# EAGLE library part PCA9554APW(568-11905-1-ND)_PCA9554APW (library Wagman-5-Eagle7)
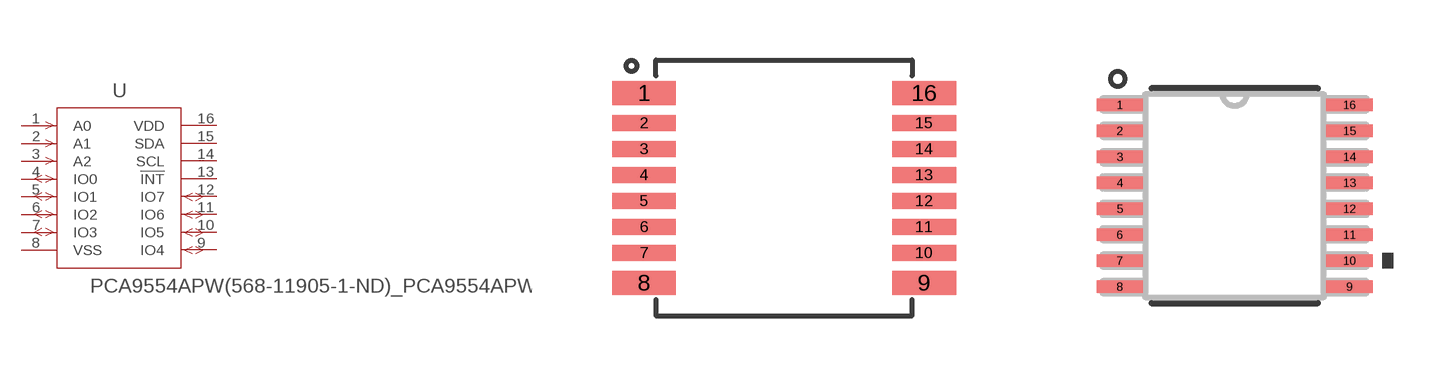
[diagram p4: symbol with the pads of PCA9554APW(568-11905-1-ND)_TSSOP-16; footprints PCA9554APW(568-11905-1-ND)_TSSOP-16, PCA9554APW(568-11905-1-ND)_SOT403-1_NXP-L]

Designator prefix U

## PCA9554APW(568-11905-1-ND)_PCA9554APW (BUILT_BY: EMA_UL_Team; MANUFACTURER_PART_NUMBER: PCA9554APW; SOURCELIBRARY: NXP_2011-11-10; VENDOR: NXP)  [PCA9554APW(568-11905-1-ND)_TSSOP-16]
1  A0  in
2  A1  in
3  A2  in
4  IO0
5  IO1
6  IO2
7  IO3
8  VSS  pwr
9  IO4
10  IO5
11  IO6
12  IO7
13  !INT  pas
14  SCL  pas
15  SDA  pas
16  VDD  pwr

## PCA9554APW(568-11905-1-ND)_PCA9554APWSOT403-1_NXP-L (BUILT_BY: EMA_UL_Team; MANUFACTURER_PART_NUMBER: PCA9554APW; SOURCELIBRARY: NXP_2011-11-10; VENDOR: NXP)  [PCA9554APW(568-11905-1-ND)_SOT403-1_NXP-L]
Pads as for PCA9554APW(568-11905-1-ND)_TSSOP-16

## PCA9554APW(568-11905-1-ND)_PCA9554APWSOT403-1_NXP-M (BUILT_BY: EMA_UL_Team; MANUFACTURER_PART_NUMBER: PCA9554APW; SOURCELIBRARY: NXP_2011-11-10; VENDOR: NXP)  [PCA9554APW(568-11905-1-ND)_SOT403-1_NXP-M]
Pads as for PCA9554APW(568-11905-1-ND)_TSSOP-16

## Footprint PCA9554APW(568-11905-1-ND)_TSSOP-16 (pad centres in mm)
smd 1.6 x 0.6: 1 -3.5,2.375; 8 -3.5,-2.375; 9 3.5,-2.375; 16 3.5,2.375
smd 1.6 x 0.4: 2 -3.5,1.625; 3 -3.5,0.975; 4 -3.5,0.325; 5 -3.5,-0.325; 6 -3.5,-0.975; 7 -3.5,-1.625; 10 3.5,-1.625; 11 3.5,-0.975; 12 3.5,-0.325; 13 3.5,0.325; 14 3.5,0.975; 15 3.5,1.625

## Footprint PCA9554APW(568-11905-1-ND)_SOT403-1_NXP-L (pad centres in mm)
smd 1.162 x 0.305: 1 -2.871,2.275; 2 -2.871,1.625; 3 -2.871,0.975; 4 -2.871,0.325; 5 -2.871,-0.325; 6 -2.871,-0.975; 7 -2.871,-1.625; 8 -2.871,-2.275; 9 2.871,-2.275; 10 2.871,-1.625; 11 2.871,-0.975; 12 2.871,-0.325; 13 2.871,0.325; 14 2.871,0.975; 15 2.871,1.625; 16 2.871,2.275

## Footprint PCA9554APW(568-11905-1-ND)_SOT403-1_NXP-M (pad centres in mm)
smd 1.762 x 0.355: 1 -2.971,2.275; 2 -2.971,1.625; 3 -2.971,0.975; 4 -2.971,0.325; 5 -2.971,-0.325; 6 -2.971,-0.975; 7 -2.971,-1.625; 8 -2.971,-2.275; 9 2.971,-2.275; 10 2.971,-1.625; 11 2.971,-0.975; 12 2.971,-0.325; 13 2.971,0.325; 14 2.971,0.975; 15 2.971,1.625; 16 2.971,2.275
